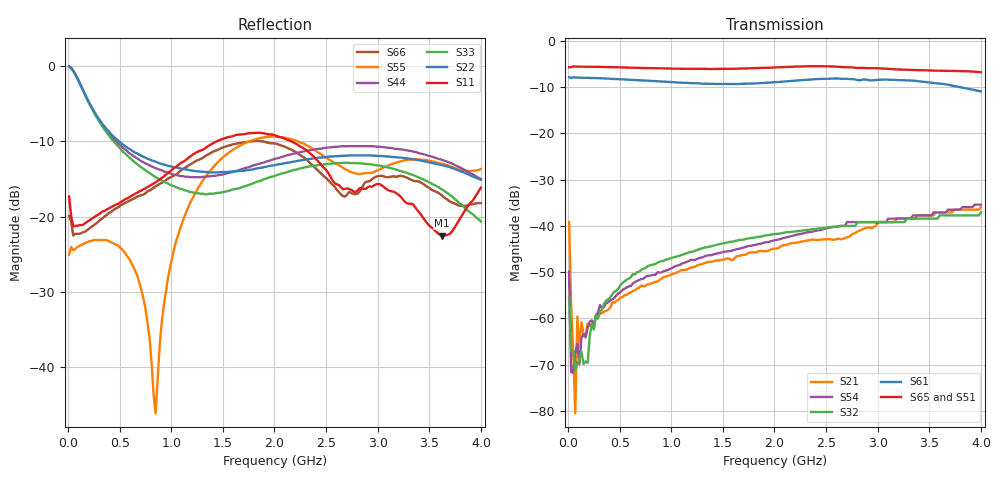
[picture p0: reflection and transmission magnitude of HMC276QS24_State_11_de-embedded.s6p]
! Hittite Microwave Corporation
! 20 Alpha Road
! Chelmsford, MA 01824
! Tel: 978-250-3343
! Fax: 978-250-3373
! Device: HMC276QS24, 0.7-3.0 GHz, GaAS MMIC 4x2 Switch Matrix in 24-lead QSOP package
! Misc: Data was de-embedded to package pins.
!  Port 1 = OP1
!  Port 2 = VL
!  Port 3 = VH
!  Port 4 = HH
!  Port 5 = HL
!  Port 6 = OP2
!  Vdd = +5 V
!  Vctl = 0 V[Logic 0] / +5 V[Logic 1]
!  State 11,  HL to OP1,  HL to OP2
!  Control Lines (Logic)
!  HV 1 = 1, Tone 1 = 0
!  HV 2 = 1, Tone 2 = 0
!  Data reformated to new Touchstone file format - Wed Jan 10 15:54:05 2007
# MHz S DB R 50
! 6 Port Network Data
! freq  dbS11  angS11  dbS12  angS12  dbS13  angS13  dbS14  angS14
!  dbS15  angS15  dbS16  angS16
!  dbS21  angS21  dbS22  angS22
!  dbS23  angS23  dbS24  angS24  dbS25  angS25  dbS26  angS26
!  dbS31  angS31  dbS32  angS32  dbS33  angS33  dbS34  angS34
!  dbS35  angS35  dbS36  angS36
!  dbS41  angS41  dbS42  angS42
!  dbS43  angS43  dbS44  angS44  dbS45  angS45  dbS46  angS46
!  dbS51  angS51  dbS52  angS52  dbS53  angS53  dbS54  angS54
!  dbS55  angS55  dbS56  angS56
!  dbS61  angS61  dbS62  angS62
!  dbS63  angS63  dbS64  angS64  dbS65  angS65  dbS66  angS66
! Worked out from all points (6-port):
!   201 points, 10 MHz to 4 GHz, reference 50 ohm
!   strongest paths, dB at 10 MHz, 1.008 GHz, 2.005 GHz, 3.002 GHz, 4 GHz:
!     S65: -5.7, -6.0, -5.7, -6.0, -6.8
!     S51: -5.8, -6.3, -6.0, -6.0, -6.8
!     S61: -7.9, -8.9, -9.0, -8.4, -10.9
!     S32: -55.5, -46.9, -41.8, -39.2, -37.1
!     S54: -49.9, -49.1, -43.1, -39.2, -35.4
!     S21: -39.2, -50.4, -44.9, -39.2, -35.9
!   lowest |S11| = -22.5 dB at 3.621 GHz (marker M1), VSWR 1.16, Z = 50.6 + j7.54 ohm
!   |S11| at or under -10 dB: start of sweep to 1.439 GHz; 2.163 GHz to end of sweep
